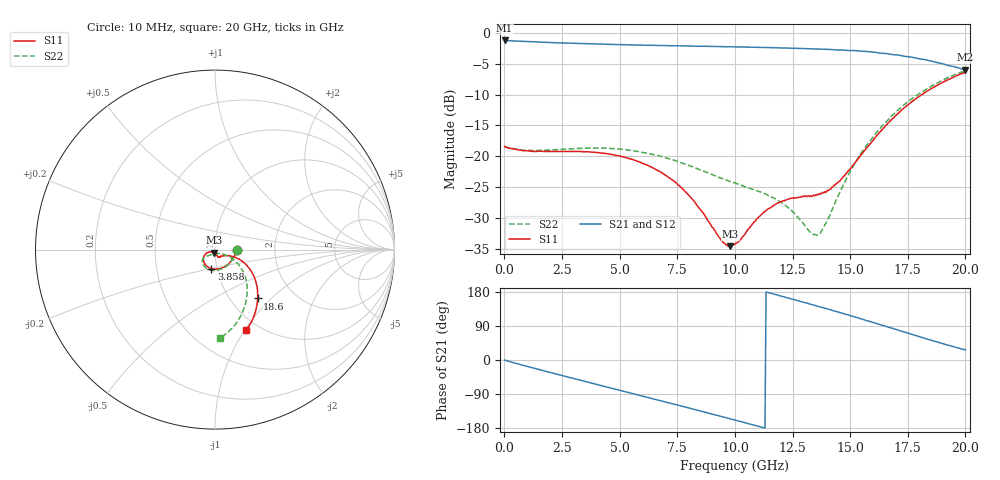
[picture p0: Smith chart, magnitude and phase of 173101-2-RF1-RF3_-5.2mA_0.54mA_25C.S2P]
!  2-Port S-parameters saved by WinCal
! VAR MeasName=S-Parameters (CALIBRATED_DATA) read from VNA (N5242A)
! VAR MeasDate=2017-7-20 9:26:01
! VAR NAME=173101-2-RF1-RF3_-5.2mA_0.54mA_25C
! VAR FILENAME=173101-2-RF1-RF3_-5.2mA_0.54mA_25C.S2P
! VAR DATE=2017-7-20 9:26:01
! VAR PHYS_PORTS=1,2
# Hz S DB R 50
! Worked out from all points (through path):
!   401 points, 10 MHz to 20 GHz, reference 50 ohm
!   highest |S21| = -1.20 dB at 10 MHz (marker M1); lowest = -6.0 dB at 20 GHz (marker M2)
!   group delay of S21, straight-line fit = 45.9 ps
!   lowest |S11| = -34.6 dB at 9.805 GHz (marker M3), VSWR 1.04, Z = 49.2 - j1.69 ohm
!   |S11| at or under -10 dB: start of sweep to 18.1 GHz
!   |S22| runs from -32.8 to -6.1 dB; largest |S21 - S12| = 0.0076
!   S11 on the Smith chart (normalised r, x): 10 MHz: 1.27, -0.00; 3.858 GHz: 0.94, -0.20; 18.6 GHz: 1.33, -0.83; 20 GHz: 0.87, -1.01
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1e7  -18.41 -0.5  -1.20 -0.3  -1.20 -0.3  -18.37 -0.5
1.559225e9  -19.18 -48.7  -1.48 -26.1  -1.48 -26.1  -19.04 -47.6
3.358325e9  -19.25 -90.9  -1.71 -54.4  -1.71 -54.4  -18.70 -87.4
3.858075e9  -19.34 -100.9  -1.77 -62.2  -1.77 -62.1  -18.65 -96.4
5.357325e9  -20.31 -127.3  -1.91 -85.4  -1.92 -85.3  -18.99 -119.1
6.70665e9  -22.39 -146.5  -2.01 -106.4  -2.00 -106.3  -19.92 -134.2
7.956025e9  -26.16 -157.5  -2.09 -125.9  -2.11 -125.8  -21.42 -142.8
9.4053e9  -33.65 -135.7  -2.21 -148.9  -2.20 -148.8  -23.55 -144.1
9.8051e9  -34.59 -113.2  -2.23 -155.3  -2.22 -155.2  -24.11 -143.0
1.0005e10  -34.27 -101.5  -2.25 -158.5  -2.25 -158.5  -24.32 -142.2
1.105448e10  -29.79 -72.3  -2.32 -175.5  -2.33 -175.4  -25.73 -137.6
1.175412e10  -27.82 -69.0  -2.38 172.9  -2.39 173.1  -26.88 -133.7
1.245378e10  -26.84 -66.9  -2.46 161.3  -2.45 161.4  -28.79 -126.7
1.335332e10  -26.51 -57.8  -2.57 146.1  -2.55 146.2  -32.56 -94.5
1.36032e10  -26.11 -53.3  -2.59 141.8  -2.59 141.8  -32.70 -76.3
1.38031e10  -25.85 -48.4  -2.65 138.3  -2.65 138.4  -31.82 -59.6
1.455272e10  -24.06 -31.8  -2.73 125.5  -2.73 125.6  -25.91 -29.8
1.525238e10  -20.85 -22.9  -2.88 112.8  -2.86 113.1  -20.84 -26.5
1.670165e10  -14.44 -25.7  -3.40 85.9  -3.44 85.9  -13.86 -38.7
1.76012e10  -11.38 -35.5  -3.88 69.4  -3.87 69.6  -10.88 -51.0
1.86007e10  -8.84 -48.8  -4.64 50.6  -4.67 51.0  -8.46 -65.8
2e10  -6.36 -68.8  -5.96 26.5  -6.00 27.1  -6.12 -86.8
